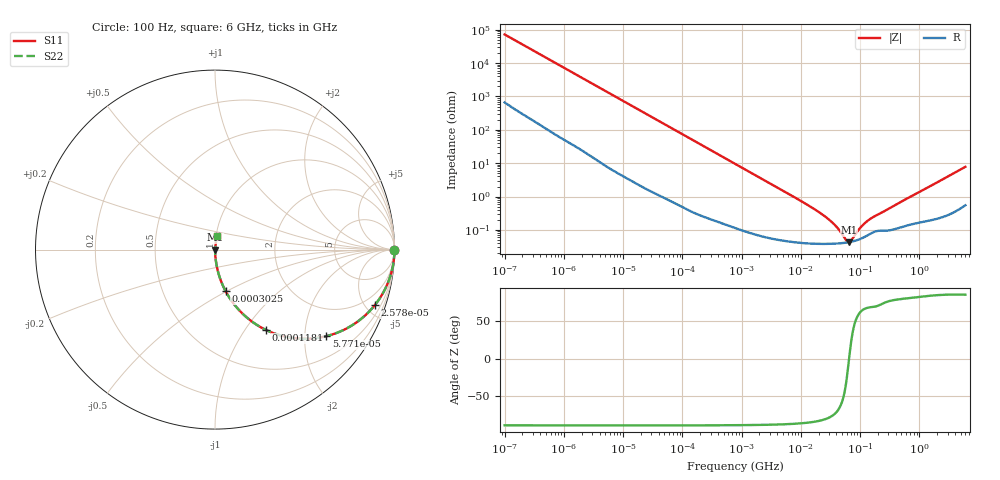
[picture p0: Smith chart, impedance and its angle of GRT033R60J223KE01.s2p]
!Murata Part Number: GRT033R60J223KE01
!These Parameters are Measured in Series Mode Connection
!Data Generated on Jun 19, 2026
!  o--ll--o
!Port1  Port2
!  o------o
!Operation Temp=25[degC], DC Bias Voltage=0[V]
!Freq. Start=100[Hz] Stop=6[GHz] 401[Steps]
# Hz S RI R 50
!Freq.(Hz) S11(Real) S11(Imag) S21(Real) S21(Imag) S12(Real) S12(Imag) S22(Real) S22(Imag)
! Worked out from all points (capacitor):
!   401 points, 100 Hz to 6 GHz, reference 50 ohm
!   read as one part in series: C = 22 nF near 109 Hz
!   lowest |Z| = 43.1 mohm at 65.19 MHz (marker M1)
!   series resonance near 65.29 MHz, so ESL is about 270 pH
!   S11 on the Smith chart (normalised r, x): 100 Hz: open; 25.78 kHz: 1.03, -5.73; 57.71 kHz: 1.02, -2.57; 118.1 kHz: 1.01, -1.26; 302.5 kHz: 1.00, -0.49; 6 GHz: 1.01, +0.16
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100  1 -0.00139  1.47e-05 0.00139  1.47e-05 0.00139  1 -0.00139
2008  0.9991 -0.0274  0.000936 0.0274  0.000936 0.0274  0.9991 -0.0274
8416  0.9865 -0.1128  0.0135 0.1128  0.0135 0.1128  0.9865 -0.1128
25777  0.8899 -0.3102  0.1101 0.3102  0.1101 0.3102  0.8899 -0.3102
40335  0.7692 -0.4184  0.2308 0.4184  0.2308 0.4184  0.7692 -0.4184
57709  0.6212 -0.482  0.3788 0.482  0.3788 0.482  0.6212 -0.482
82567  0.4466 -0.4939  0.5534 0.4939  0.5534 0.4939  0.4466 -0.4939
118133  0.2843 -0.4478  0.7157 0.4478  0.7157 0.4478  0.2843 -0.4478
184852  0.141 -0.3444  0.859 0.3444  0.859 0.3444  0.141 -0.3444
302498  0.0589 -0.2312  0.9411 0.2312  0.9411 0.2312  0.0589 -0.2312
774597  0.0104 -0.0955  0.9896 0.0955  0.9896 0.0955  0.0104 -0.0955
2481164  0.00153 -0.0303  0.9985 0.0303  0.9985 0.0303  0.00153 -0.0303
1.555665e7  0.000409 -0.00461  0.9996 0.00461  0.9996 0.00461  0.000409 -0.00461
3.330331e7  0.000388 -0.00169  0.9996 0.00169  0.9996 0.00169  0.000388 -0.00169
4.35672e7  0.000396 -0.000967  0.9996 0.000967  0.9996 0.000967  0.000396 -0.000967
5.699437e7  0.000415 -0.000317  0.9996 0.000317  0.9996 0.000317  0.000415 -0.000317
6.518806e7  0.000431 -3.7e-06  0.9996 3.7e-06  0.9996 3.7e-06  0.000431 -3.7e-06
7.129496e7  0.000445 0.000204  0.9996 -0.000204  0.9996 -0.000204  0.000445 0.000204
9.753859e7  0.000525 0.000948  0.9995 -0.000948  0.9995 -0.000948  0.000525 0.000948
1.275994e8  0.00066 0.00162  0.9993 -0.00162  0.9993 -0.00162  0.00066 0.00162
3.124326e8  0.000991 0.00435  0.999 -0.00435  0.999 -0.00435  0.000991 0.00435
6e9  0.0114 0.0765  0.9886 -0.0765  0.9886 -0.0765  0.0114 0.0765
